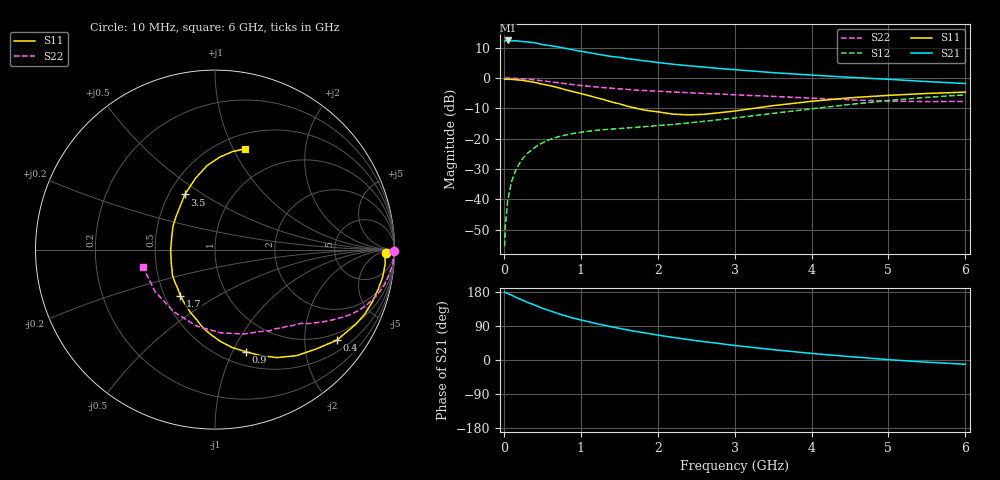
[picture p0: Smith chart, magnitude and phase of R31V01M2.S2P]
! SIEMENS Small Signal Semiconductors
! BFR181
! Si NPN RF Bipolar Junction Transistor in SOT23
! VCE = 1 V  IC = 1.2 mA
! Common Emitter S-Parameters:  May  1996
# GHz  S  MA  R  50
!  f  S11  S21  S12  S22
! GHz  MAG  ANG  MAG  ANG  MAG  ANG  MAG  ANG
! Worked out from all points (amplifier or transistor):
!   36 points, 10 MHz to 6 GHz, reference 50 ohm
!   highest |S21| = 12.3 dB at 50 MHz (marker M1)
!   |S21| within 3 dB of that: start of sweep to 883.2 MHz
!   unconditionally stable (mu >= 1): 1.801 GHz to 3.796 GHz
!   at 250 MHz: K = 0.18, MSG = 19.2 dB, |S12| = -26.4 dB
!   at 1.4 GHz: K = 0.84, MSG = 12.0 dB, |S12| = -16.8 dB
!   at 6 GHz: K = 0.91, MSG = 1.9 dB, |S12| = -5.6 dB
!   S11 on the Smith chart (normalised r, x): 10 MHz: 36, -13; 400 MHz: 0.79, -2.82; 900 MHz: 0.64, -1.13; 1.7 GHz: 0.60, -0.34; 3.5 GHz: 0.60, +0.42; 6 GHz: 0.65, +1.11
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0.01  0.9526 -1.0  4.053 179.4  0.0017 95.7  0.9985 -0.5
0.02  0.9459 -1.9  4.082 178.1  0.0036 85.7  0.9947 -1.0
0.05  0.9517 -4.6  4.142 175.6  0.0096 86.8  0.9959 -2.3
0.1  0.9471 -9.2  4.068 171.3  0.0196 83.4  0.994 -4.5
0.15  0.9347 -14.0  4.098 165.9  0.0294 80.0  0.9849 -6.9
0.3  0.8882 -27.9  3.929 152.7  0.0564 72.8  0.9563 -13.1
0.4  0.8462 -36.6  3.798 145.0  0.0715 67.5  0.9276 -17.0
0.5  0.7911 -44.3  3.551 136.6  0.0854 62.9  0.8968 -20.3
0.7  0.6947 -60.0  3.255 123.0  0.1068 55.6  0.8356 -25.7
0.9  0.5949 -73.1  2.904 110.6  0.1217 50.3  0.7761 -29.9
1.1  0.5141 -86.4  2.62 101.0  0.1324 46.7  0.7305 -33.2
1.2  0.4752 -92.6  2.491 96.0  0.137 45.3  0.7113 -34.8
1.4  0.4021 -104.9  2.258 87.5  0.1438 43.7  0.677 -37.4
1.7  0.3213 -127.1  2.009 75.9  0.1527 43.8  0.6321 -40.5
2  0.2769 -148.8  1.795 65.8  0.1647 44.2  0.6068 -44.1
2.2  0.2534 -164.6  1.684 59.6  0.1718 45.3  0.587 -46.8
2.6  0.2516 162.9  1.51 48.4  0.1933 47.1  0.5552 -52.5
3  0.2851 139.5  1.369 38.3  0.219 48.3  0.5275 -59.5
3.5  0.35 118.7  1.223 27.3  0.2612 48.0  0.4969 -71.1
4.5  0.4713 95.2  1.023 8.9  0.3665 42.0  0.4373 -104.1
5.5  0.5553 79.8  0.872 -5.7  0.4789 29.7  0.4078 -145.0
6  0.5844 73.5  0.809 -11.3  0.5276 22.2  0.4117 -166.0
